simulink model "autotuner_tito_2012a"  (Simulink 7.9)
settings: Solver=ode3  StartTime=0.0  StopTime=simopt.Tf  FixedStep=simopt.h  RelTol=1e-3
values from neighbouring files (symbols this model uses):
  params = []    [setParams.m]
  simopt = []    [setParams.m]
libraries: simulink x2

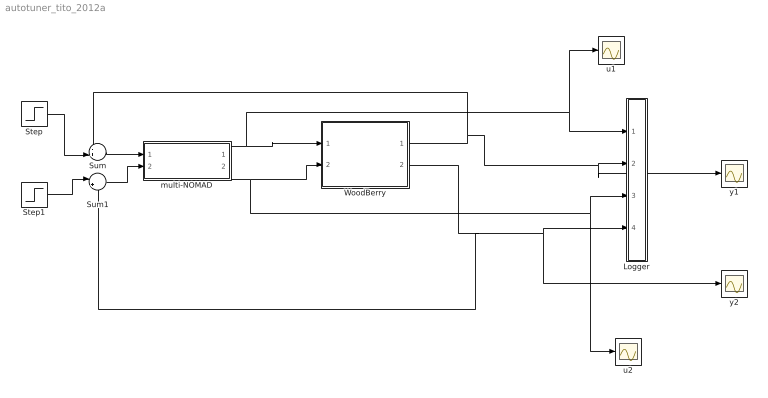
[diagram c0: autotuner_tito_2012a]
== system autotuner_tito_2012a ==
  Logger : Subsystem
  Step : Step  Time=0  After=0  SampleTime=simopt.h
  Step1 : Step  Time=0  After=0  SampleTime=simopt.h
  Sum : Sum  Inputs=-+|
  Sum1 : Sum  Inputs=|+-
  WoodBerry : Subsystem
  multi-NOMAD : Subsystem
  u1 : Scope
  u2 : Scope
  y1 : Scope
  y2 : Scope
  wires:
  multi-NOMAD/1(u1) -> Logger/1(u1), u1/1, WoodBerry/1(u1)
  multi-NOMAD/2(u2) -> Logger/3(u2), u2/1, WoodBerry/2(u2)
  WoodBerry/1(y1) -> Logger/2(y1), y1/1, Sum/1
  WoodBerry/2(y2) -> Logger/4(y2), y2/1, Sum1/2
  Step/1 -> Sum/2
  Step1/1 -> Sum1/1
  Sum/1 -> multi-NOMAD/1(e1)
  Sum1/1 -> multi-NOMAD/2(e2)

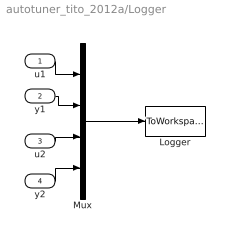
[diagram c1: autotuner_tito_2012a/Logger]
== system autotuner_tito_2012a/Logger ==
  u1 : Inport  SampleTime=simopt.h
  y1 : Inport  Port=2  SampleTime=simopt.h
  u2 : Inport  Port=3  SampleTime=simopt.h
  y2 : Inport  Port=4  SampleTime=simopt.h
  Logger : ToWorkspace  VariableName=simout  SampleTime=simopt.h  SaveFormat=Structure With Time
  Mux : Mux
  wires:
  Mux/1 -> Logger/1
  u1/1 -> Mux/1
  y1/1 -> Mux/2
  u2/1 -> Mux/3
  y2/1 -> Mux/4

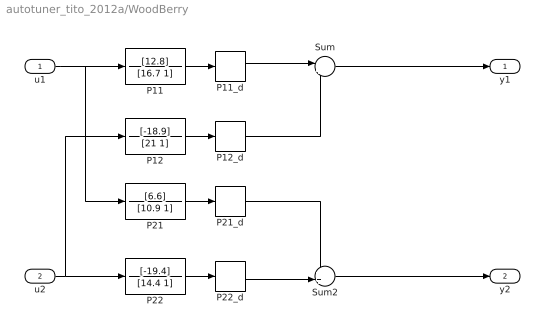
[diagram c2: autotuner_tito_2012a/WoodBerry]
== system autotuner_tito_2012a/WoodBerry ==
  u1 : Inport
  u2 : Inport  Port=2
  P11 : TransferFcn  Numerator=[12.8]  Denominator=[16.7 1]
  P11_d : TransportDelay
  P12 : TransferFcn  Numerator=[-18.9]  Denominator=[21 1]
  P12_d : TransportDelay  DelayTime=3
  P21 : TransferFcn  Numerator=[6.6]  Denominator=[10.9 1]
  P21_d : TransportDelay  DelayTime=7
  P22 : TransferFcn  Numerator=[-19.4]  Denominator=[14.4 1]
  P22_d : TransportDelay  DelayTime=3
  Sum : Sum  Inputs=|++
  Sum2 : Sum  Inputs=++|
  y1 : Outport
  y2 : Outport  Port=2
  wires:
  Sum2/1 -> y2/1
  P22_d/1 -> Sum2/2
  P22/1 -> P22_d/1
  P21_d/1 -> Sum2/1
  P21/1 -> P21_d/1
  u2/1 -> P22/1, P12/1
  P12_d/1 -> Sum/2
  P12/1 -> P12_d/1
  u1/1 -> P21/1, P11/1
  Sum/1 -> y1/1
  P11_d/1 -> Sum/1
  P11/1 -> P11_d/1

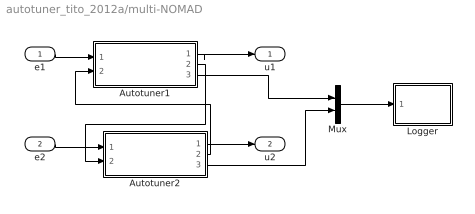
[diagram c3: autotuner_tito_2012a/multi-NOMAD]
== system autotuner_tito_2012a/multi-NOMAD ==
  e1 : Inport
  e2 : Inport  Port=2
  Autotuner1 : Subsystem
  Autotuner2 : Subsystem
  Logger : Subsystem
  Mux : Mux  Inputs=2
  u1 : Outport
  u2 : Outport  Port=2
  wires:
  Mux/1 -> Logger/1(result)
  Autotuner2/3(result2) -> Mux/2
  Autotuner1/3(result1) -> Mux/1
  e2/1 -> Autotuner2/1(e)
  e1/1 -> Autotuner1/1(e)
  Autotuner2/1(u) -> u2/1
  Autotuner1/1(u) -> u1/1
  Autotuner2/2(done) -> Autotuner1/2(other_done)
  Autotuner1/2(done) -> Autotuner2/2(other_done)

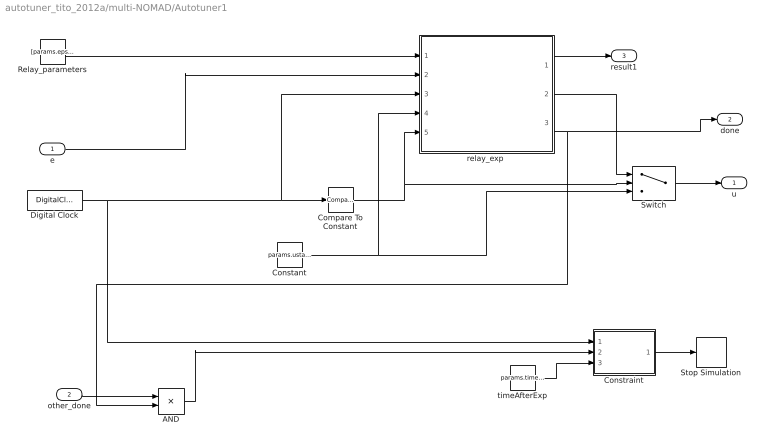
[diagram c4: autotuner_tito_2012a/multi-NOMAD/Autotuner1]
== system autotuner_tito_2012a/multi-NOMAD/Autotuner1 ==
  e : Inport
  other_done : Inport  Port=2
  AND : Product
  Compare To Constant : simulink/Logic and Bit Operations/Compare To Constant  relop=>=  const=params.expStartTime  OutDataTypeStr=boolean
  Constant : Constant  Value=params.ustart  SampleTime=simopt.h
  Constraint : MATLAB Function  TreatAsAtomicUnit=on  SystemSampleTime=simopt.h
  Digital Clock : DigitalClock  SampleTime=simopt.h
  Relay_parameters : Constant  Value=[params.eps, params.gamma, simopt.h, params.low_limit, params.dev_limit, 1 , params.uon, params.hyst, params.noiseMeasureTime, 1, params.gamma2, params.switches, params.ystep, params.ustep]  SampleTime=simopt.h
  Stop Simulation : Stop
  Switch : Switch  Criteria=u2 ~= 0
  "relay_exp " : MATLAB Function  TreatAsAtomicUnit=on  SystemSampleTime=simopt.h
  timeAfterExp : Constant  Value=params.timeAfterExp
  u : Outport
  done : Outport  Port=2
  result1 : Outport  Port=3
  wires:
  "relay_exp "/1(result) -> result1/1
  timeAfterExp/1 -> Constraint/3(timeAfterExp)
  "relay_exp "/3(done) -> done/1, AND/2
  other_done/1 -> AND/1
  AND/1 -> Constraint/2(all_done)
  Constraint/1(stop) -> Stop Simulation/1
  Digital Clock/1 -> Constraint/1(time), Compare To Constant/1, "relay_exp "/3(t)
  e/1 -> "relay_exp "/2(e)
  Constant/1 -> Switch/3, "relay_exp "/4(u_ref)
  Compare To Constant/1 -> "relay_exp "/5(run_exp), Switch/2
  "relay_exp "/2(u) -> Switch/1
  Relay_parameters/1 -> "relay_exp "/1(relay_par)
  Switch/1 -> u/1

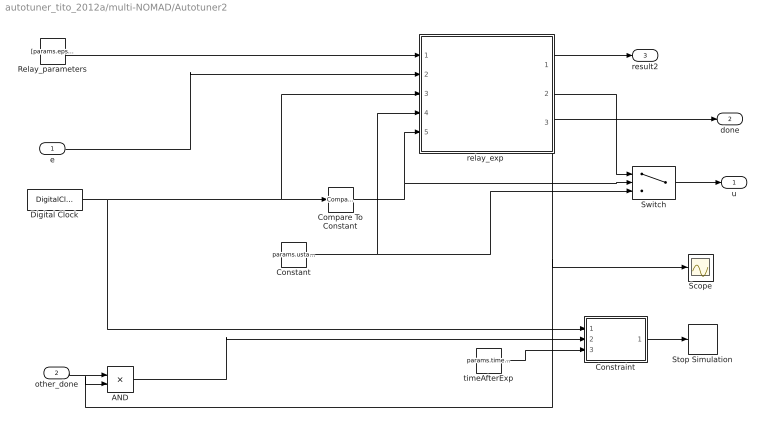
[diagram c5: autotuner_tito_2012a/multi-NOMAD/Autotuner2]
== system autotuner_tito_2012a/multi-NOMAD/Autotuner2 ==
  e : Inport
  other_done : Inport  Port=2
  AND : Product
  Compare To Constant : simulink/Logic and Bit Operations/Compare To Constant  relop=>=  const=params.expStartTime  OutDataTypeStr=boolean
  Constant : Constant  Value=params.ustart  SampleTime=simopt.h
  Constraint : MATLAB Function  TreatAsAtomicUnit=on  SystemSampleTime=simopt.h
  Digital Clock : DigitalClock  SampleTime=simopt.h
  Relay_parameters : Constant  Value=[params.eps,params.gamma, simopt.h,params.low_limit,params.dev_limit,1,params.uon,params.hyst,params.noiseMeasureTime,1,params.gamma2,params.switches,params.ystep,params.ustep]  SampleTime=simopt.h
  Scope : Scope
  Stop Simulation : Stop
  Switch : Switch  Criteria=u2 ~= 0
  "relay_exp " : MATLAB Function  TreatAsAtomicUnit=on  SystemSampleTime=simopt.h
  timeAfterExp : Constant  Value=params.timeAfterExp
  u : Outport
  done : Outport  Port=2
  result2 : Outport  Port=3
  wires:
  Digital Clock/1 -> Constraint/1(time), Compare To Constant/1, "relay_exp "/3(t)
  Constant/1 -> Switch/3, "relay_exp "/4(u_ref)
  Compare To Constant/1 -> "relay_exp "/5(run_exp), Switch/2
  timeAfterExp/1 -> Constraint/3(timeAfterExp)
  "relay_exp "/3(done) -> done/1, AND/2, Scope/1
  other_done/1 -> AND/1
  AND/1 -> Constraint/2(all_done)
  Constraint/1(stop) -> Stop Simulation/1
  "relay_exp "/1(result) -> result2/1
  e/1 -> "relay_exp "/2(e)
  "relay_exp "/2(u) -> Switch/1
  Relay_parameters/1 -> "relay_exp "/1(relay_par)
  Switch/1 -> u/1

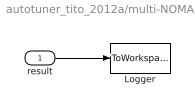
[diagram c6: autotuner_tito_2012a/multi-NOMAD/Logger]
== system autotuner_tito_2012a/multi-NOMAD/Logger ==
  result : Inport  SampleTime=simopt.h
  Logger : ToWorkspace  VariableName=result  SampleTime=simopt.h  SaveFormat=Structure With Time
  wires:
  result/1 -> Logger/1

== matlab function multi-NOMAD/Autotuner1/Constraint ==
%function stop = Constraint(tstop, time, done)
function stop = Constraint(time, all_done, timeAfterExp)
%#codegen
persistent tstopp first
if isempty(tstopp)
    tstopp = 10000;
    first = true;
end
if all_done == 1 && first 
    tstopp = time;
    first = false;
end
if time > tstopp+timeAfterExp;
    stop = 1;
else
    stop = 0;
end

== matlab function multi-NOMAD/Autotuner1/relay_exp
 ==
function [result, u, done]= relay_exp(relay_par, e,t, u_ref, run_exp)


%%%%%%%%%% Definitions and default values %%%%%%%%%%%%%%
y = -e;
% Relay parameters, values from workspace.
persistent d1 d2 u_on u_off h
gamma = relay_par(11); % index 2 is gamma, 11 is gamma2 
t_sample = relay_par(3);
bigYup = relay_par(6);
relayMaxDev = relay_par(7);
def_h = relay_par(8);
noiseMeasureTime = relay_par(9);
maxSwitches = relay_par(12);
ystep = relay_par(13);
ustep = relay_par(14);

persistent yref uref
if isempty(d2)
    h=def_h; % these values will be re-assigned later and never used.
    d1 = gamma;
    d2 = 1;
    u_on =  d1;
    u_off = -d2;
    uref = 0;
    yref = 0;
end

persistent u_old resultvec
if isempty(u_old)
    u_old = uref;
    resultvec = zeros(23,1);
end

persistent sample
if isempty(sample)
    sample = 0;
end

persistent startup Ksign
if isempty(Ksign)
    Ksign = 1; % Is re-assigned during at the startup phase
end

persistent param done_per
if isempty(param)
    param = [1.1, 16, 0]; % Quadtank minfas (should be an input somehow if existing PID parameters are used to bring it to its working point)
    done_per = 0;
end
PID_param = param;
done = done_per;

% To handle switches
persistent switching_times switch_index 
if isempty(switching_times)
    switching_times = zeros(1,20); % Shouldn't need to be so large
    switch_index = 1;
end

%%%%%%%%% Startup  params %%%%%%%%%%%
persistent a b c tff exp_t yh yl measureNoise first
if isempty(startup)
    tff = 5/t_sample; % According to Tore about 3-5s is appropriate for the startup growth 
    b = 40;
    c = relayMaxDev/(b-1);
    a = uref-c;
    measureNoise = 1;
    startup = 0;
    yh = 0;
    yl = 0;
    first = true;
end
%%%%%%%%%%%%%%%%%%%%%%%%%%%%%%%%%%%%%%%%%%%%%%%

result = resultvec;
if run_exp == 0
    u = 0;
    PID_param = param;
    return
end

%%%%%%%%%%%%% Program running %%%%%%%%%%%%%%%%%
sample = sample+1;

%%%%%%%%% Startup %%%%%%%%%%%%
if measureNoise == 1
    if first 
        uref = u_ref;
        yref = y;
        first = false;
        yh = yref;
        yl = yref;
    end
    u = uref;
    if sample < noiseMeasureTime/t_sample
        yh = max(yh,y);
        yl = min(yl,y);
    else
        noise = (yh-yl)/2;
        yref = (yh+yl)/2;
        %yref = y; % Could test the latest value instead of average?
        resultvec(15) = yref;
        resultvec(16) = uref;
        h = max(2*noise, def_h);
        measureNoise = 0;
        startup = 1;
        resultvec(23) = t;
    end
elseif startup == 1
    exp_t = sample-noiseMeasureTime/t_sample;
    a = uref-c;
        u = a+c*b^(exp_t/tff);
        if u > relayMaxDev+uref
            u = relayMaxDev+uref;
        end
        if exp_t > 1
            ydev = y-yref; 
            if abs(ydev) > h % outside hysteresis, stop startup and decide Ksign
                Ksign = ydev/abs(ydev);
                if bigYup == 1
                    d1 = min(relayMaxDev, gamma*abs(u-uref));
                    d2 = d1/gamma;
                else
                    d2 = min(relayMaxDev, gamma*abs(u-uref));
                    d1 = d2/gamma;
                end
                startup = 0;
            elseif exp_t > tff
                u = uref+relayMaxDev;
            end
        end
elseif run_exp == 1
    %%%%%% Update amplitudes %%%%%%%
    u_on = uref+Ksign*d1;
    u_off = uref-Ksign*d2;
    %%%%%% Calculate new u %%%%%%%%%
    u = rel_func(y,u_old,u_on, u_off,yref,h);
else 
    u = 0; %Shouldn't be needed?
end

%%%%%%% At switching points %%%%%%%
if sample>1 && (u-uref)*(u_old-uref) < 0
    switching_times(switch_index) = t;
    if switch_index > 2
        tp = switching_times(switch_index)-switching_times(switch_index-2);
        resultvec(19) = tp;
    end
    if switch_index == 3 % Step in yref/uref after two switches
        yref = yref+ystep*h;
        uref = uref+(d1+d2)/2*Ksign*ustep;
    end
    if switch_index > maxSwitches
        done_per = 1;
        resultvec(17) = t;
    end
    switch_index = switch_index+1;
end
%%%% store data %%%%%%
u_old = u;
end

function u = rel_func(y,uold,uon,uoff,yref,h)
  if y <= yref-h
    u = uon;
  elseif y < yref+h && y > yref-h
    u = uold;
  else u = uoff;
  end
end

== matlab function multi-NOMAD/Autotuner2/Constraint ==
%function stop = Constraint(tstop, time, done)
function stop = Constraint(time, all_done, timeAfterExp)
%#codegen
persistent tstopp first
if isempty(tstopp)
    tstopp = 10000;
    first = true;
end
if all_done == 1 && first 
    tstopp = time;
    first = false;
end
if time > tstopp+timeAfterExp;
    stop = 1;
else
    stop = 0;
end

== matlab function multi-NOMAD/Autotuner2/relay_exp
 ==
function [result, u, done]= relay_exp(relay_par, e,t, u_ref, run_exp)


%%%%%%%%%% Definitions and default values %%%%%%%%%%%%%%
y = -e;
% Relay parameters, values from workspace.
persistent d1 d2 u_on u_off h
gamma = relay_par(2); % index 2 is gamma, 11 is gamma2 
t_sample = relay_par(3);
bigYup = relay_par(6);
relayMaxDev = relay_par(7);
def_h = relay_par(8);
noiseMeasureTime = relay_par(9);
maxSwitches = relay_par(12);
ystep = relay_par(13);
ustep = relay_par(14);

persistent yref uref
if isempty(d2)
    h=def_h; % these values will be re-assigned later and never used. 
    d1 = gamma;
    d2 = 1;
    u_on =  d1;
    u_off = -d2;
    uref = 0;
    yref = 0;
end

persistent u_old resultvec
if isempty(u_old)
    u_old = uref;
    resultvec = zeros(23,1);
end

persistent sample
if isempty(sample)
    sample = 0;
end

persistent startup Ksign
if isempty(Ksign)
    Ksign = 1;  % Is re-assigned during at the startup phase
end

persistent param done_per
if isempty(param)
    param = [1.1, 16, 0]; % Quadtank minfas (should be an input somehow if existing PID parameters are used to bring it to its working point)
    done_per = 0;
end
PID_param = param;
done = done_per;

% To handle switches
persistent switching_times switch_index 
if isempty(switching_times)
    switching_times = zeros(1,20);
    switch_index = 1;
end

%%%%%%%%% Startup  params %%%%%%%%%%%
persistent a b c tff exp_t yh yl measureNoise first
if isempty(startup)
    tff = 5/t_sample; % According to Tore about 3-5s is appropriate for the startup growth 
    b = 40;
    c = relayMaxDev/(b-1);
    a = uref-c;
    measureNoise = 1;
    startup = 0;
    yh = 0;
    yl = 0;
    first = true;
end
%%%%%%%%%%%%%%%%%%%%%%%%%%%%%%%%%%%%%%%%%%%%%%%

result = resultvec;
if run_exp == 0
    u = 0;
    PID_param = param;
    return
end

%%%%%%%%%%%%% Program running %%%%%%%%%%%%%%%%%
sample = sample+1;

%%%%%%%%% Startup %%%%%%%%%%%%
if measureNoise == 1
    if first 
        uref = u_ref;
        yref = y;
        first = false;
        yh = yref;
        yl = yref;
    end
    u = uref;
    if sample < noiseMeasureTime/t_sample
        yh = max(yh,y);
        yl = min(yl,y);
    else
        noise = (yh-yl)/2;
        yref = (yh+yl)/2;
        %yref = y; % Could test the latest value instead of average?
        resultvec(15) = yref;
        resultvec(16) = uref;
        h = max(2*noise, def_h);
        measureNoise = 0;
        startup = 1;
        resultvec(23) = t;
    end
elseif startup == 1
    exp_t = sample-noiseMeasureTime/t_sample;
    a = uref-c;
        u = a+c*b^(exp_t/tff);
        if u > relayMaxDev+uref
            u = relayMaxDev+uref;
        end
        if exp_t > 1
            ydev = y-yref; 
            if abs(ydev) > h % outside hysteresis, stop startup and decide Ksign
                Ksign = ydev/abs(ydev);
                if bigYup == 1
                    d1 = min(relayMaxDev, gamma*abs(u-uref));
                    d2 = d1/gamma;
                else
                    d2 = min(relayMaxDev, gamma*abs(u-uref));
                    d1 = d2/gamma;
                end
                startup = 0;
            elseif exp_t > tff
                u = uref+relayMaxDev;
            end
        end
elseif run_exp == 1
    %%%%%% Update amplitudes %%%%%%%
    u_on = uref+Ksign*d1;
    u_off = uref-Ksign*d2;
    %%%%%% Calculate new u %%%%%%%%%
    u = rel_func(y,u_old,u_on, u_off,yref,h);
else 
    u = 0; % Shouldn't be needed?
end

%%%%%%% At switching points %%%%%%%
if sample>1 && (u-uref)*(u_old-uref) < 0
    switching_times(switch_index) = t;
    if switch_index > 2
        tp = switching_times(switch_index)-switching_times(switch_index-2);
        resultvec(19) = tp;
    end
    if switch_index == 3 % Step in yref/uref after two switches
        yref = yref+ystep*h;
        uref = uref+(d1+d2)/2*Ksign*ustep;
    end
    if switch_index > maxSwitches
        done_per = 1;
        resultvec(17) = t;
    end
    switch_index = switch_index+1;
end
%%%% store data %%%%%%
u_old = u;
end

function u = rel_func(y,uold,uon,uoff,yref,h)
  if y <= yref-h
    u = uon;
  elseif y < yref+h && y > yref-h
    u = uold;
  else u = uoff;
  end
end
